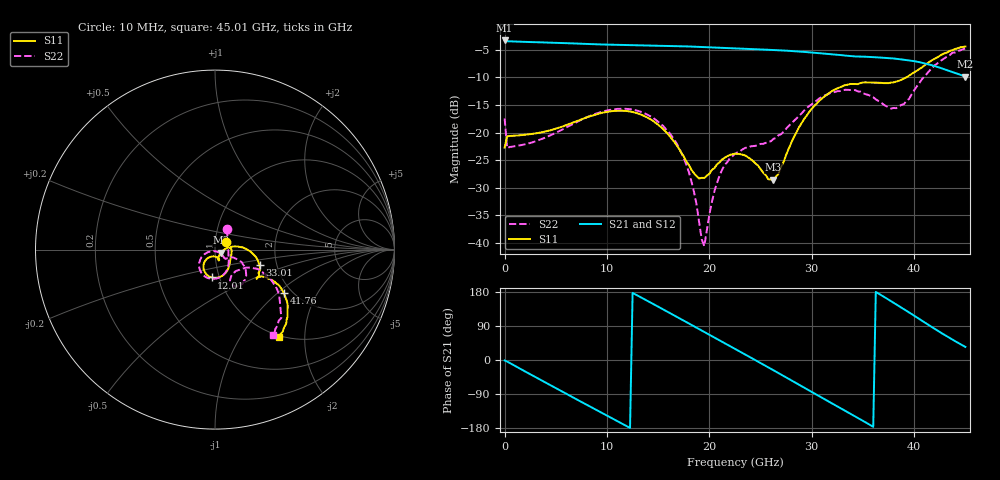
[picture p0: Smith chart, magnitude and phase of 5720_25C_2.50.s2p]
! Device:  ADRF5720
! Description: 0.5dB LSB GaAs MMIC 6-bit Digital Attenuator
! Frequency:  0.000009 -  40 GHz
! Ports:
!	RF1	= Port 1
!	RF2	= Port 2
! Vdd:  3.3 Volt
! Vss:  -3.3 Volt
! Control:  0/3.3 Volt
! State:  2.50 dB attenuation
! Data:  The device was measured using G-S-G Probes on a matrix board.
!  Data was collected using an calibrated 4 port network analyzer.
!  The reference plane for this measurement is at the launchers.
! Note:  Analog Devices supplies this data as a sample of measured data
!  for this product.  Your particular data for this product may vary.
!  Data was taken at 25 degrees C.
!  Analog Devices reserves the right to change this data at anytime.
# GHZ S DB R 45.0
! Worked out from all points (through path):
!   181 points, 10 MHz to 45.01 GHz, reference 45 ohm
!   highest |S21| = -3.31 dB at 10 MHz (marker M1); lowest = -9.8 dB at 45.01 GHz (marker M2)
!   group delay of S21, straight-line fit = 42 ps
!   lowest |S11| = -28.6 dB at 26.26 GHz (marker M3), VSWR 1.08, Z = 48 - j1.71 ohm
!   |S11| at or under -10 dB: start of sweep to 39.27 GHz
!   |S22| runs from -40.6 to -4.8 dB; largest |S21 - S12| = 0.00078
!   S11 on the Smith chart (normalised r, x): 10 MHz: 1.12, +0.10; 12.01 GHz: 0.92, -0.29; 33.01 GHz: 1.62, -0.30; 41.76 GHz: 1.81, -1.10; 45.01 GHz: 0.97, -1.49
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0.01  -22.74 36.2  -3.31 -1.2  -3.31 -1.2  -17.45 59.5
0.26  -20.71 0.4  -3.45 -4.1  -3.46 -4.1  -22.81 1.2
4.26  -19.70 -34.8  -3.70 -63.2  -3.70 -63.2  -20.70 -34.3
7.76  -17.44 -58.8  -3.92 -114.2  -3.92 -114.2  -17.46 -61.2
10.01  -16.25 -78.2  -4.06 -146.8  -4.06 -146.8  -16.01 -82.3
12.01  -16.12 -97.0  -4.16 -175.7  -4.16 -175.6  -15.73 -103.0
15.26  -18.99 -124.9  -4.27 137.0  -4.27 137.0  -18.42 -137.6
16.76  -22.20 -131.4  -4.34 114.9  -4.34 114.9  -21.81 -151.6
18.01  -25.92 -124.9  -4.40 96.3  -4.40 96.3  -27.19 -160.3
19.51  -28.24 -89.3  -4.50 74.0  -4.50 74.0  -40.61 -84.0
20.26  -26.76 -74.4  -4.56 62.8  -4.56 62.9  -32.53 -38.5
21.01  -25.39 -68.7  -4.62 51.7  -4.61 51.7  -27.76 -35.1
22.76  -23.87 -70.0  -4.76 25.6  -4.76 25.7  -23.59 -40.7
26.26  -28.58 -28.6  -5.04 -26.9  -5.04 -26.9  -21.16 -30.9
28.26  -20.85 9.7  -5.25 -57.5  -5.25 -57.5  -17.90 -23.5
30.26  -15.17 1.2  -5.54 -88.3  -5.54 -88.3  -14.49 -29.7
33.01  -11.60 -19.4  -5.99 -130.2  -6.00 -130.2  -12.38 -48.6
35.51  -10.94 -33.0  -6.29 -168.5  -6.29 -168.4  -13.18 -63.6
37.76  -10.95 -33.3  -6.55 155.2  -6.55 155.2  -15.66 -52.5
40.01  -9.08 -28.0  -7.06 116.8  -7.06 116.9  -12.35 -25.6
41.76  -6.88 -32.3  -7.81 86.6  -7.81 86.6  -8.33 -30.6
45.01  -4.40 -54.0  -9.85 34.5  -9.85 34.6  -4.79 -55.8
